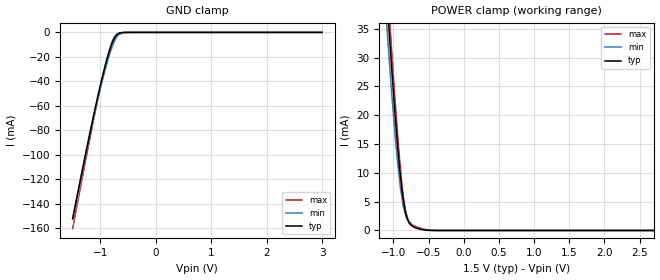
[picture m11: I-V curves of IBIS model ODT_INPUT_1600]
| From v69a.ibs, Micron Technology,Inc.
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| MODEL ODT_INPUT_1600 (ODT Input Model, 1600Mbps)
[Model]   ODT_INPUT_1600
Model_type   Input
Vinl = 600.000mV
Vinh = 900.000mV
|   typ   min   max
C_comp   0.58pF   0.48pF   0.68pF
[Model Spec]
| Input threshold voltage corners
Vinl   0.6000V   0.5625V   0.6375V
Vinh   0.9000V   0.8625V   0.9375V
[Receiver Thresholds]
Vth   =  0.750V
Vth_min  =  0.735V
Vth_max  =  0.765V
Vinh_ac  =  0.150V
Vinh_dc  =  0.100V
Vinl_ac  = -0.150V
Vinl_dc  = -0.100V
Tslew_ac =  10.00ns |Not specified, so set to high value
[Voltage Range]   1.5000V   1.4250V   1.5750V
| Junction Temperature (Ambient temp is 35C typ, 95C min, 0C max)
[Temperature Range]   50.0   110.0   0.0
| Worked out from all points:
|   GND clamp passes 1 mA (typ) near -0.67 V on its own axis
|   POWER clamp passes 1 mA (typ) near -0.75 V on its own axis
[GND Clamp]
|   Voltage   I(typ)   I(min)   I(max)
-1.5V     -152.2mA   -152.2mA   -160.3mA
-1.195V   -83.57mA   -84.89mA   -88.17mA
-1.09V    -61.23mA   -63.26mA   -64.37mA
-980mV    -39.42mA   -42.22mA   -40.73mA
-875mV    -21.01mA   -24.3mA    -20.55mA
-830mV    -14.22mA   -17.55mA   -13.26mA
-790mV    -9.108mA   -12.26mA   -7.847mA
-750mV    -5.075mA   -7.616mA   -3.982mA
-710mV    -2.343mA   -4.146mA   -1.761mA
-625mV    -287.8uA   -738.9uA   -221.3uA
-505mV    -8.053uA   -42.81uA   -5.048uA
3V        0A         0A         0A
[POWER Clamp]
|   Voltage   I(typ)   I(min)   I(max)
-1.5V     121.2mA    114.2mA    127.2mA
-1.09V    39.96mA    34.96mA    43.5mA
-1.07V    36.29mA    31.5mA     39.66mA
-1.055V   33.59mA    28.95mA    36.82mA
-1.045V   31.8mA     27.29mA    34.93mA
-940mV    14.59mA    11.76mA    16.63mA
-875mV    6.616mA    5.443mA    7.478mA
-830mV    3.216mA    2.88mA     3.545mA
-790mV    1.706mA    1.661mA    1.793mA
-730mV    716uA      851uA      984.8uA
-410mV    3.061uA    11.47uA    8.872uA
3V        0A         0A         0A
